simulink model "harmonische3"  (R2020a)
settings: Solver=ode45  StartTime=-8  StopTime=8  MaxStep=0.01  RelTol=1e-3  EnableMultiTasking=on

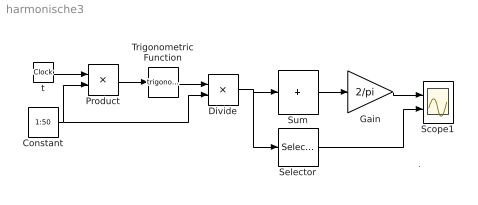
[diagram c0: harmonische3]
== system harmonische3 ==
  note: .
  Constant : Constant  Value=1:50
  Divide : Product  Inputs=*/
  Gain : Gain  Gain=2/pi  SaturateOnIntegerOverflow=on
  Product : Product  RndMeth=Zero
  Scope1 : Scope  NumInputPorts=2
  Selector : Selector  IndexOptions=Index vector (dialog)  Indices=1:5  OutputSizes=1
  Sum : Sum  Inputs=+  SaturateOnIntegerOverflow=on
  Trigonometric Function : Trigonometry
  t : Clock
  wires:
  Sum/1 -> Gain/1
  Divide/1 -> Sum/1, Selector/1
  Gain/1 -> Scope1/1
  t/1 -> Product/1
  Constant/1 -> Product/2, Divide/2
  Product/1 -> Trigonometric Function/1
  Trigonometric Function/1 -> Divide/1
  Selector/1 -> Scope1/2
